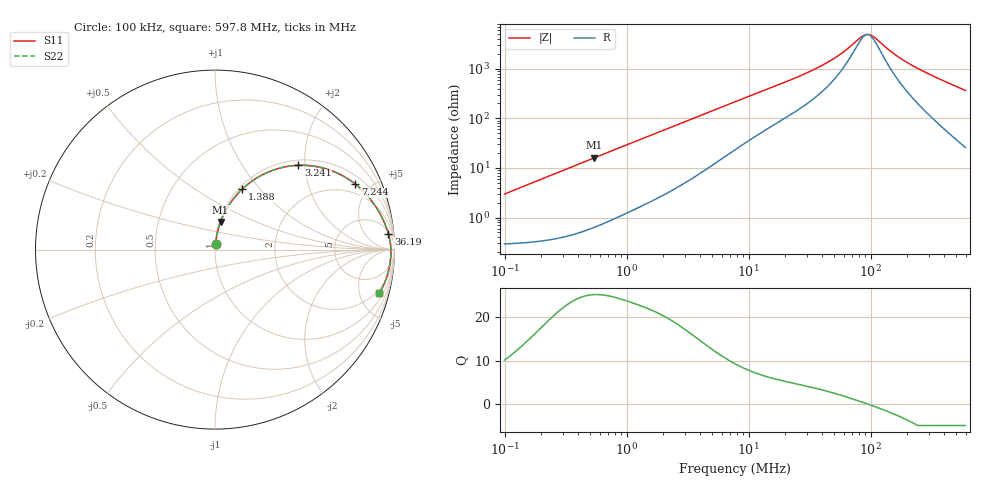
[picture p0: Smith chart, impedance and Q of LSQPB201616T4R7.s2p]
! LSQPB201616T4R7  S-PARAMETER MODEL  ( General Type )
! Model Generated by TAIYO YUDEN Corporation (http://www.ty-top.com)
! Version 2.0
! TAIYO YUDEN Control No. 100810NC14SB-FKC
! Copyright(c) 2008 TAIYO YUDEN CO.,LTD. All Rights Reserved.
! Product Description (link to TY-COMPAS)
! https://ds.yuden.co.jp/TYCOMPAS/or/detail?pn=LSQPB201616T4R7M&u=M
! Products Name : Inductors
! Characteristics :
!  Inductance : 4.7 uH , SRF(min) : 78 MHz , DC Resistance(max) : 0.351 Ohm
!  Rated Current : Saturation :660 mA , Temp Rise : 610 mA (40 degC)
!  Case Size : 2.0 x 1.6 / 0.079 x 0.063 [mm/inch] , Thickness : 1.6 / 0.063 [mm/inch]
!  (Conditions: Temperature = 25 degC , DC Bias Current/Voltage = 0A / 0V)
! External Node Assignments :
!  1  o---GGG---o  2
! GND o---------o GND
! Frequency Range : 0.1MHz  -  597.797849MHz  [ 402 STEP ]
# MHz S RI R 50
! Freq[MHz].  S11 Real  S11 Imag  S21 Real  S21 Imag  S12 Real  S12 Imag  S22 Real  S22 Imag
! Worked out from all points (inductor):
!   401 points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, 100 kHz to 597.8 MHz, reference 50 ohm
!   read as one part in series: L = 4.72 uH near 104.4 kHz
!   highest Q = 25.3 at 545 kHz (marker M1), where L = 4.69 uH
!   self-resonance near 93.78 MHz
!   S11 on the Smith chart (normalised r, x): 100 kHz: 1.01, +0.06; 1.388 MHz: 1.04, +0.80; 3.241 MHz: 1.11, +1.85; 7.244 MHz: 1.42, +4.05; 36.19 MHz: 7, +20; 597.8 MHz: 1.52, -7.34
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0.1  0.0038 0.0295  0.9962 -0.0295  0.9962 -0.0295  0.0038 0.0295
0.223528  0.0078 0.0655  0.9922 -0.0655  0.9922 -0.0655  0.0078 0.0655
0.429114  0.0207 0.1235  0.9793 -0.1235  0.9793 -0.1235  0.0207 0.1235
0.54504  0.031 0.1546  0.969 -0.1546  0.969 -0.1546  0.031 0.1546
0.918378  0.0761 0.2452  0.9239 -0.2452  0.9239 -0.2452  0.0761 0.2452
1.388058  0.1504 0.3358  0.8496 -0.3358  0.8496 -0.3358  0.1504 0.3358
1.84139  0.231 0.3982  0.769 -0.3982  0.769 -0.3982  0.231 0.3982
3.240572  0.4644 0.4694  0.5356 -0.4694  0.5356 -0.4694  0.4644 0.4694
4.588639  0.6213 0.4491  0.3787 -0.4491  0.3787 -0.4491  0.6213 0.4491
7.243576  0.7827 0.3641  0.2173 -0.3641  0.2173 -0.3641  0.7827 0.3641
7.731739  0.8002 0.3496  0.1998 -0.3496  0.1998 -0.3496  0.8002 0.3496
14.21137  0.9068 0.2215  0.0932 -0.2215  0.0932 -0.2215  0.9068 0.2215
33.17799  0.9636 0.0973  0.0364 -0.0973  0.0364 -0.0973  0.9636 0.0973
36.19225  0.9665 0.0876  0.0335 -0.0876  0.0335 -0.0876  0.9665 0.0876
53.52547  0.9754 0.0483  0.0246 -0.0483  0.0246 -0.0483  0.9754 0.0483
82.67767  0.9797 0.0105  0.0203 -0.0105  0.0203 -0.0105  0.9797 0.0105
92.17118  0.9801 0.00144  0.0199 -0.00144  0.0199 -0.00144  0.9801 0.00144
105.0131  0.9803 -0.00945  0.0197 0.00945  0.0197 0.00945  0.9803 -0.00945
142.3714  0.9795 -0.0359  0.0205 0.0359  0.0205 0.0359  0.9795 -0.0359
184.8075  0.9773 -0.0611  0.0227 0.0611  0.0227 0.0611  0.9773 -0.0611
250.5526  0.9719 -0.0954  0.0281 0.0954  0.0281 0.0954  0.9719 -0.0954
597.7978  0.9164 -0.2437  0.0836 0.2437  0.0836 0.2437  0.9164 -0.2437
